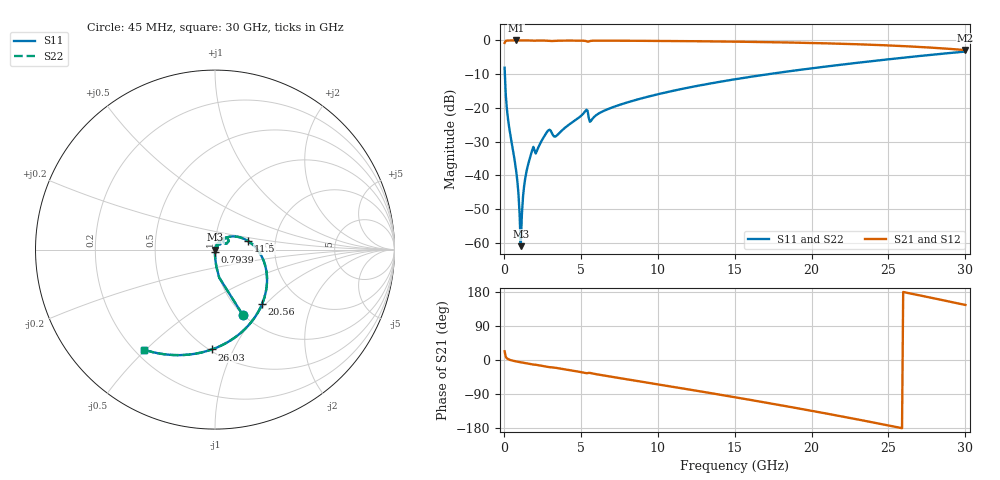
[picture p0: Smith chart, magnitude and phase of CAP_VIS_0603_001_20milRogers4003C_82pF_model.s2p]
! S-parameter model data by Modelithics Inc.  support@modelithics.com  813-866-6335  Tampa FL USA
! S-Parameter data specifications:
! Substrate: 20-mil Rogers 4003C, substrate thickness, H=0.508mm, Dielectric constant, Er=3.75
! PCB Mounting Pad Footprint: Pad width, PadW=0.90mm , Pad length, PadL=1.00mm , Pad gap, PadG (edge-to-edge)=1.00mm , Reference planes=3.0mm apart
! Created Wed Nov 18 13:30:40 2015
# hz S ma R 50
! 2 Port Network Data from SP1.SP block
! freq  magS11  angS11  magS21  angS21  magS12  angS12  magS22  angS22
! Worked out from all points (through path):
!   401 points, 45 MHz to 30 GHz, reference 50 ohm
!   highest |S21| = -0.01 dB at 793.9 MHz (marker M1); lowest = -2.9 dB at 30 GHz (marker M2)
!   group delay of S21, straight-line fit = 19.8 ps
!   lowest |S11| = -61.1 dB at 1.093 GHz (marker M3), VSWR 1.00, Z = 50.1 - j0.0081 ohm
!   |S11| at or under -10 dB: 62.97 MHz to 17.21 GHz (17.15 GHz wide, 199 % of centre)
!   |S22| runs from -61.1 to -3.3 dB; largest |S21 - S12| = 0
!   S11 on the Smith chart (normalised r, x): 45 MHz: 1.00, -0.86; 793.9 MHz: 1.00, -0.02; 11.5 GHz: 1.44, +0.14; 20.56 GHz: 1.32, -0.95; 26.03 GHz: 0.51, -0.83; 30 GHz: 0.24, -0.49
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4.5e7  0.3942 -67.0  0.9188 23.0  0.9188 23.0  0.3942 -67.0
3.4455e8  0.05058 -88.4  0.9982 1.0  0.9982 1.0  0.05058 -88.4
7.93875e8  0.01168 -90.0  0.9991 -3.7  0.9991 -3.7  0.01168 -90.0
9.4365e8  0.005384 -86.2  0.9991 -4.9  0.9991 -4.9  0.005384 -86.2
1.093425e9  0.000886 -5.2  0.999 -6.0  0.999 -6.0  0.000886 -5.2
1.2432e9  0.004849 71.4  0.9989 -7.1  0.9989 -7.1  0.004849 71.4
1.318088e9  0.007057 74.1  0.9989 -7.7  0.9989 -7.7  0.007057 74.1
1.467862e9  0.01137 75.5  0.9987 -8.7  0.9987 -8.7  0.01137 75.5
1.8423e9  0.02373 69.6  0.9959 -11.5  0.9959 -11.5  0.02373 69.6
2.890725e9  0.04646 57.0  0.9871 -18.5  0.9871 -18.5  0.04646 57.0
3.414938e9  0.03839 55.1  0.9897 -20.9  0.9897 -20.9  0.03839 55.1
5.062462e9  0.07787 53.9  0.9914 -32.3  0.9914 -32.3  0.07787 53.9
5.287125e9  0.08931 48.0  0.9835 -34.2  0.9835 -34.2  0.08931 48.0
5.73645e9  0.06773 47.4  0.9887 -35.4  0.9887 -35.4  0.06773 47.4
1.007992e10  0.1604 24.2  0.983 -64.6  0.983 -64.6  0.1604 24.2
1.150279e10  0.1893 14.8  0.9776 -74.2  0.9776 -74.2  0.1893 14.8
1.50225e10  0.2654 -9.1  0.959 -98.3  0.959 -98.3  0.2654 -9.1
2.003996e10  0.3864 -45.0  0.9158 -134.4  0.9158 -134.4  0.3864 -45.0
2.056418e10  0.4001 -48.9  0.9098 -138.3  0.9098 -138.3  0.4001 -48.9
2.505742e10  0.5266 -83.8  0.8418 -173.3  0.8418 -173.3  0.5266 -83.8
2.603096e10  0.5563 -91.8  0.8222 178.8  0.8222 178.8  0.5563 -91.8
3e10  0.6836 -125.3  0.7191 145.2  0.7191 145.2  0.6836 -125.3
